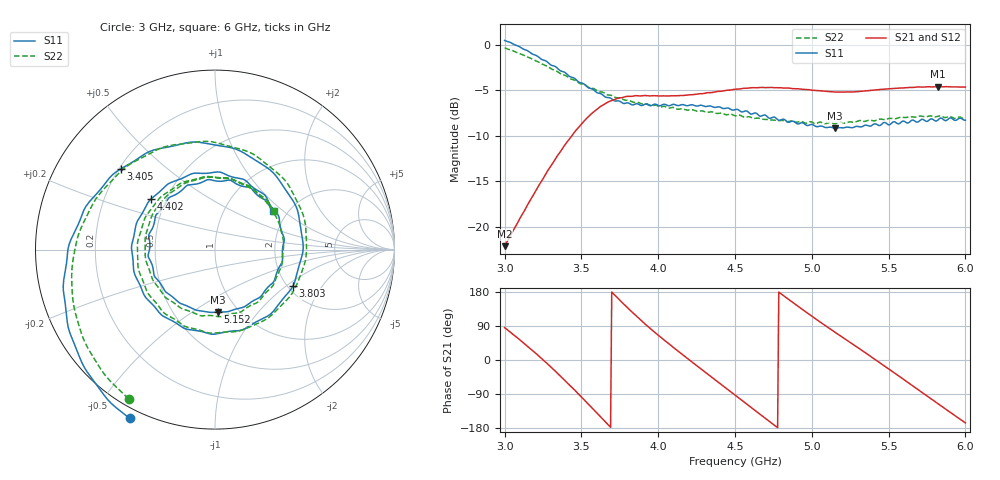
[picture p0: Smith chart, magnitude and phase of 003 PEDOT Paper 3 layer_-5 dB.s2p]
!  04/11/2025  18:48:37
! Ref Plane: 0.000 mm
# MHZ S MA R  50
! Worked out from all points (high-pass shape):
!   401 points, 3 GHz to 6 GHz, reference 50 ohm
!   highest |S21| = -4.60 dB at 5.82 GHz (marker M1); lowest = -22.1 dB at 3 GHz (marker M2)
!   |S21| within 3 dB of the highest: 3.564 GHz to end of sweep
!   lowest |S11| = -9.2 dB at 5.152 GHz (marker M3), VSWR 2.07, Z = 40.5 - j32 ohm
!   |S11| at or under -10 dB: nowhere
!   |S22| runs from -8.7 to -0.3 dB; largest |S21 - S12| = 0.014
!   S11 on the Smith chart (normalised r, x): 3 GHz: -0.04, -0.61; 3.405 GHz: 0.21, +0.36; 3.803 GHz: 2.14, -1.12; 4.402 GHz: 0.41, +0.30; 5.152 GHz: 0.81, -0.64; 6 GHz: 1.68, +0.84
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3000  1.054 -116.8  0.07859 85.4  0.07929 86.5  0.9606 -120.1
3202.5  0.8745 -165.1  0.1578 17.8  0.1581 18.7  0.8154 -168.3
3405  0.6901 139.2  0.2913 -58.8  0.293 -58.0  0.6705 134.5
3502.5  0.6158 104.8  0.3693 -98.5  0.3697 -97.9  0.6083 100.0
3577.5  0.5667 75.4  0.4263 -130.1  0.4281 -129.4  0.5755 70.4
3667.5  0.5128 35.2  0.4818 -167.9  0.4823 -167.3  0.5315 32.1
3802.5  0.4796 -24.9  0.5206 136.9  0.5225 138.0  0.4949 -26.4
3907.5  0.4687 -66.7  0.5258 97.6  0.5263 98.9  0.4723 -66.7
4005  0.4625 -99.2  0.5231 64.0  0.5232 65.0  0.4576 -99.8
4207.5  0.4665 -160.8  0.5312 -1.3  0.5343 -0.3  0.4394 -162.5
4402.5  0.4545 141.4  0.5542 -62.1  0.5564 -61.0  0.421 138.2
4500  0.44 109.8  0.5695 -92.6  0.5724 -91.6  0.4073 106.9
4612.5  0.4168 73.6  0.5807 -127.5  0.5819 -126.9  0.3962 70.2
4755  0.4008 27.7  0.5807 -171.8  0.581 -170.8  0.3856 22.7
4867.5  0.38 -7.8  0.5752 154.3  0.5747 155.4  0.3822 -13.1
5002.5  0.3647 -46.6  0.5625 114.9  0.562 115.8  0.3755 -52.7
5152.5  0.3484 -87.1  0.5496 72.8  0.5495 73.6  0.3683 -94.8
5347.5  0.3618 -139.1  0.5579 19.5  0.5589 20.3  0.3798 -146.8
5505  0.3633 176.2  0.5728 -24.8  0.575 -23.6  0.3941 170.6
5677.5  0.3777 126.4  0.5848 -74.0  0.5875 -72.8  0.4008 122.2
5820  0.3854 82.7  0.5887 -115.0  0.5914 -113.8  0.4044 82.0
6000  0.3851 33.6  0.5846 -166.1  0.5865 -165.2  0.3899 33.2
